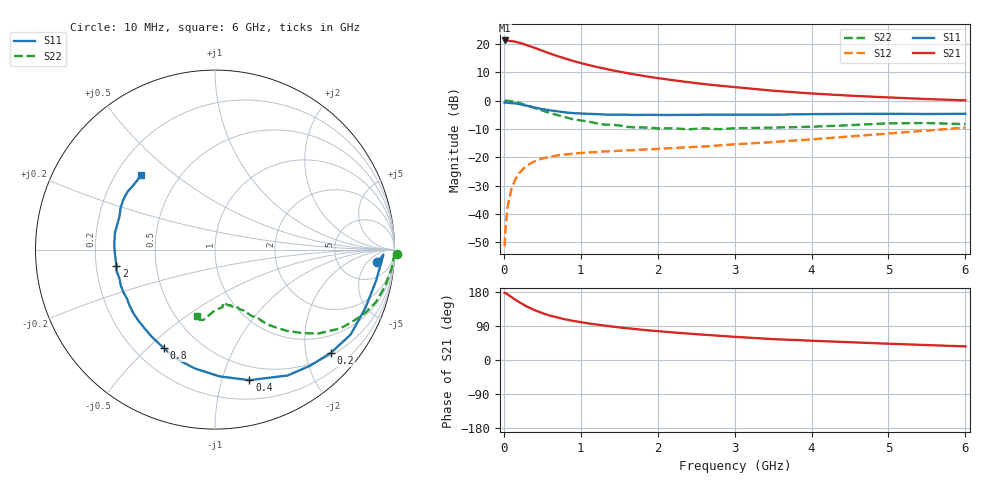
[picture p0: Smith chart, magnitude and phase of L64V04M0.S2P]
!  INFINEON TECHNOLOGIES Small Signal Semiconductors
! BFR380L3 , Si-NPN RF-Transistor in TSLP-3-1
!  Vce=4 V,  Ic=4 mA
! Common Emitter S-Parameters:  07. March 2005
#  GHz  S  MA  R  50
! f  S11  S21  S12  S22
! GHz  Mag  Ang  Mag  Ang  Mag  Ang  Mag  Ang
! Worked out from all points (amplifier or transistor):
!   36 points, 10 MHz to 6 GHz, reference 50 ohm
!   highest |S21| = 21.2 dB at 10 MHz (marker M1)
!   |S21| within 3 dB of that: start of sweep to 439.1 MHz
!   unconditionally stable (mu >= 1): 2.665 GHz to 4.615 GHz
!   at 250 MHz: K = 0.13, MSG = 22.1 dB, |S12| = -24.2 dB
!   at 1.4 GHz: K = 0.69, MSG = 14.3 dB, |S12| = -17.9 dB
!   at 6 GHz: K = 0.92, MSG = 4.8 dB, |S12| = -9.6 dB
!   S11 on the Smith chart (normalised r, x): 10 MHz: 12, -10; 200 MHz: 0.55, -2.52; 400 MHz: 0.37, -1.23; 800 MHz: 0.32, -0.56; 2 GHz: 0.29, -0.08; 6 GHz: 0.30, +0.38
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0.01  0.906 -4.5  11.48 176.8  0.0027 84.1  1.014 -1.3
0.02  0.9388 -1.7  11.42 177.3  0.0053 94.0  0.9963 -2.6
0.05  0.9143 -10.9  11.4 172.8  0.0135 85.7  0.9894 -6.1
0.1  0.899 -21.1  11.15 166.0  0.028 79.5  0.9698 -12.1
0.15  0.8918 -32.0  10.9 159.0  0.0411 73.6  0.9437 -18.0
0.2  0.8647 -41.7  10.47 152.5  0.0525 69.3  0.9089 -22.8
0.3  0.8098 -60.0  9.478 141.0  0.0715 60.3  0.8258 -32.1
0.4  0.7524 -75.2  8.506 131.5  0.0849 53.7  0.7391 -39.3
0.5  0.7067 -88.0  7.568 123.9  0.0951 48.9  0.6656 -44.2
0.6  0.671 -99.9  6.746 117.2  0.1022 45.2  0.6042 -48.5
0.7  0.6457 -109.2  6.068 112.0  0.1078 43.3  0.552 -51.9
0.8  0.618 -117.6  5.5 107.2  0.1122 41.3  0.5073 -55.1
0.9  0.6003 -125.7  5.001 103.2  0.1153 40.0  0.4677 -57.1
1.1  0.5824 -137.0  4.242 96.5  0.1215 39.1  0.4246 -60.9
1.5  0.5629 -155.0  3.241 86.0  0.1301 39.7  0.3637 -67.0
2  0.5568 -170.6  2.49 76.2  0.1404 42.7  0.3221 -74.3
2.2  0.5565 -175.0  2.285 72.7  0.1456 44.4  0.3245 -74.8
2.8  0.5639 172.6  1.833 63.9  0.1616 49.5  0.3124 -82.2
3.5  0.5628 161.4  1.49 55.1  0.1853 54.0  0.3332 -88.4
4.5  0.5815 151.9  1.22 46.9  0.2328 60.1  0.3676 -95.3
5.5  0.5788 140.9  1.063 39.4  0.2955 61.9  0.401 -102.1
6  0.5848 134.6  1.008 35.9  0.3328 61.3  0.3838 -105.3
